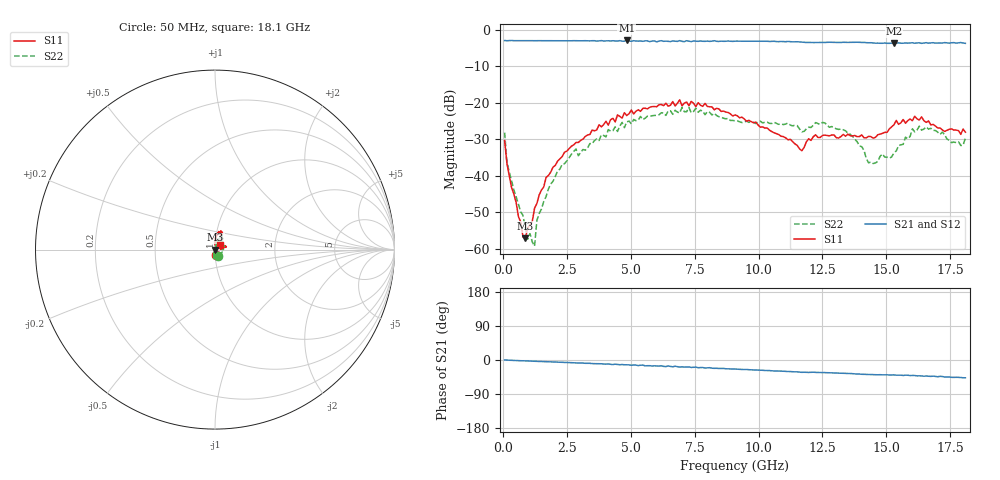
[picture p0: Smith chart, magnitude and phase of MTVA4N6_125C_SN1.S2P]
! Network Analyzer HP8720D.06.14 Serial No. US36140669
! 28 Jun 2005  14:04:03
! Frequency  S11  S21  S12  S22
# HZ  S  DB R 50
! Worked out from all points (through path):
!   201 points, 50 MHz to 18.1 GHz, reference 50 ohm
!   highest |S21| = -2.87 dB at 4.833 GHz (marker M1); lowest = -3.7 dB at 15.3 GHz (marker M2)
!   group delay of S21, straight-line fit = 7.23 ps
!   lowest |S11| = -57.2 dB at 862.2 MHz (marker M3), VSWR 1.00, Z = 50.1 - j0.0397 ohm
!   |S11| at or under -10 dB: start of sweep to end of sweep
!   |S22| runs from -59.3 to -21.3 dB; largest |S21 - S12| = 0.022
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5e7  -30.32 -81.1  -2.89 0.2  -2.88 0.1  -28.17 -63.1
1.4025e8  -36.64 -84.1  -2.93 -0.2  -2.93 -0.3  -36.09 -75.4
7.72e8  -56.86 -63.3  -2.92 -2.2  -2.91 -2.0  -50.92 -65.2
8.6225e8  -57.18 -16.6  -2.92 -2.2  -2.94 -2.3  -54.28 -101.7
1.22325e9  -48.91 27.4  -2.94 -3.2  -2.93 -3.3  -59.33 10.6
1.3135e9  -47.63 35.0  -2.93 -3.5  -2.93 -3.4  -52.26 31.8
1.855e9  -39.04 41.7  -2.94 -5.0  -2.94 -5.0  -42.27 70.5
2.7575e9  -31.52 48.2  -2.92 -7.3  -2.93 -7.2  -33.34 74.7
3.1185e9  -29.94 53.7  -2.95 -8.0  -2.97 -8.3  -32.80 81.3
4.83325e9  -23.48 66.7  -2.87 -12.6  -2.97 -13.0  -25.22 68.1
6.09675e9  -20.51 66.5  -3.05 -16.1  -2.99 -16.1  -23.28 66.5
7.27e9  -20.77 73.4  -3.07 -18.3  -3.12 -19.6  -21.27 62.2
9.075e9  -23.30 86.8  -3.06 -23.9  -3.04 -24.1  -24.89 40.2
1.169225e10  -33.14 85.1  -3.33 -32.5  -3.34 -32.5  -27.95 34.8
1.21435e10  -29.28 74.8  -3.44 -32.2  -3.40 -32.5  -26.14 49.7
1.3407e10  -29.15 34.0  -3.39 -35.2  -3.37 -35.4  -27.66 45.5
1.43095e10  -29.17 2.4  -3.50 -38.5  -3.45 -38.8  -36.45 37.8
1.512175e10  -27.14 20.0  -3.66 -39.6  -3.58 -39.5  -35.21 44.5
1.530225e10  -26.01 14.3  -3.68 -39.3  -3.59 -40.3  -33.75 49.3
1.6295e10  -24.70 12.2  -3.52 -41.8  -3.51 -43.3  -26.39 1.8
1.79195e10  -28.64 48.1  -3.44 -46.4  -3.36 -45.7  -31.70 -65.8
1.81e10  -28.04 43.9  -3.66 -46.9  -3.64 -47.7  -29.66 -79.7
